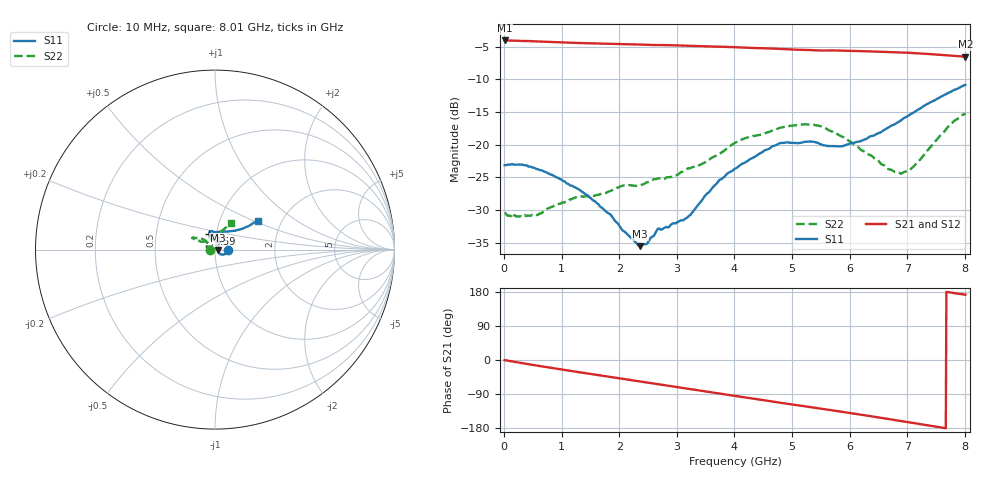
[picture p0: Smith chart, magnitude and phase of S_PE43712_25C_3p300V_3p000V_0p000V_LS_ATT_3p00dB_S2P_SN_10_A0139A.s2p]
! DEVICE ID: PE43712
! File Path: z:\PE43713\PE43713_CHAR_NOM_04292014\AMB\3p300\LS_ATT_3p00dB\PE43713_AMB_3p300V_3p000V_0p000V_LS_ATT_3p00dB_S2P_SN_10_A0139A.s2p
! Serial: 10
! Lot: A0139A
! Temp: 25C
! VDD: 3.300
! VSS: 0.000
! Control_Hi: 3.000
! Control_Lo: 0.000
! Attenuation Step: 3.00dB
! Port 1: RF1
! Port 2: RF2
! ThroughPath:1-2
! IDD: 0.0001470054
! ISS: -1.893e-007
#  Hz  S  RI  R  50
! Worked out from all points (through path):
!   801 points, 10 MHz to 8.01 GHz, reference 50 ohm
!   highest |S21| = -4.06 dB at 10 MHz (marker M1); lowest = -6.6 dB at 8.01 GHz (marker M2)
!   group delay of S21, straight-line fit = 64.3 ps
!   lowest |S11| = -35.5 dB at 2.36 GHz (marker M3), VSWR 1.03, Z = 51.7 - j0.21 ohm
!   |S11| at or under -10 dB: start of sweep to end of sweep
!   |S22| runs from -31.2 to -15.2 dB; largest |S21 - S12| = 0.0018
!   S11 on the Smith chart (normalised r, x): 10 MHz: 1.15, -0.00; 4.59 GHz: 0.92, +0.16; 8.01 GHz: 1.51, +0.53
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1e7  0.0697 -0.000317  0.6266 -0.00341  0.6264 -0.00345  -0.03 5.99e-05
1.3e8  0.0709 -0.00497  0.6238 -0.0385  0.6236 -0.0384  -0.0283 -0.000128
5.5e8  0.0621 -0.0215  0.5973 -0.152  0.597 -0.1521  -0.0286 -0.00475
1.35e9  0.0344 -0.0271  0.5003 -0.3287  0.5002 -0.3286  -0.0402 -0.00191
1.84e9  0.0233 -0.0181  0.4207 -0.4144  0.4206 -0.4143  -0.0434 0.00835
2.08e9  0.0179 -0.0125  0.3765 -0.4507  0.3765 -0.4504  -0.0469 0.0137
2.36e9  0.0167 -0.00203  0.3207 -0.4869  0.3207 -0.4867  -0.0438 0.0221
2.48e9  0.0173 0.00252  0.2957 -0.5  0.2957 -0.4999  -0.0432 0.0282
2.68e9  0.019 0.0127  0.2545 -0.5183  0.2546 -0.5183  -0.039 0.0394
3.2e9  0.00766 0.0273  0.138 -0.554  0.1382 -0.5541  -0.0486 0.0447
3.72e9  -0.00219 0.0525  0.0202 -0.5613  0.0201 -0.5612  -0.0635 0.0558
4.01e9  -0.0133 0.0642  -0.0461 -0.5547  -0.0459 -0.5547  -0.0823 0.0627
4.59e9  -0.0319 0.087  -0.1681 -0.5186  -0.168 -0.5188  -0.107 0.0644
4.81e9  -0.0306 0.0985  -0.2118 -0.4967  -0.2113 -0.4969  -0.1179 0.0661
5.35e9  -0.0203 0.1035  -0.3031 -0.4326  -0.3029 -0.4322  -0.1275 0.0649
5.86e9  0.00839 0.0968  -0.3804 -0.3611  -0.3797 -0.3611  -0.1027 0.0535
6.25e9  0.0449 0.0995  -0.4278 -0.2931  -0.4266 -0.2927  -0.0773 0.0443
6.68e9  0.0894 0.1026  -0.466 -0.2088  -0.4656 -0.2087  -0.0454 0.0462
6.89e9  0.112 0.1047  -0.4794 -0.1655  -0.4789 -0.1656  -0.028 0.0534
7.04e9  0.1286 0.11  -0.486 -0.1337  -0.4855 -0.1337  -0.0137 0.0625
7.72e9  0.2051 0.1423  -0.4818 0.01  -0.4815 0.00945  0.0612 0.1243
8.01e9  0.2372 0.1613  -0.4662 0.0623  -0.465 0.0615  0.0871 0.1498
